FUNCTION_BLOCK Example29_recoveryaccident	//any number of flyways and xbots (real physical, with at least 1 xbot having suffered a tracking error) - GetAllAccidentXbots, RecoverAccidentXbot
VAR_INPUT
	Execute : BOOL;
END_VAR
VAR_OUTPUT
	Done : BOOL;
END_VAR
VAR_IN_OUT
	PM_Controller : PMControllerType;	// the planar motor controller to use
END_VAR
VAR
	PMC_ReadNumAccidentXbots1 : PMC_ReadNumAccidentXbots;
	PMC_GetAllAccidentXbots1 : PMC_GetAllAccidentXbots;
	PMC_RecoverAccidentXbot1 : PMC_RecoverAccidentXbot;
	xbot_index : INT := 0;
	recovering_xbots : BOOL := FALSE;
	num_accident : USINT;
END_VAR

//any number of flyways and xbots (real physical, with at least 1 xbot having suffered a tracking error) - GetAllAccidentXbots, RecoverAccidentXbot

//reset index
IF(Execute = FALSE)THEN
	xbot_index := 0;
	recovering_xbots := 0;
	Done := 0;
END_IF;

//wait until a xbot has suffered a tracking error
PMC_ReadNumAccidentXbots1(Enable := Execute,nXbots => num_accident,PM_Controller := PM_Controller);
IF(num_accident > 0)THEN
	recovering_xbots := TRUE;
END_IF;

//get IDs of all xbots that have suffered tracking errors
PMC_GetAllAccidentXbots1(Execute := recovering_xbots,PM_Controller := PM_Controller);

//recover one of the accident xbots
PMC_RecoverAccidentXbot1(Execute := PMC_GetAllAccidentXbots1.Done,XbotID := PMC_GetAllAccidentXbots1.XbotIDs[xbot_index],RecoveryMode := 0,ShortAxis := 0,PM_Controller := PM_Controller);

//reset recover_accident function block and increment the index if it is done and not all accident xbots have been recovered 
IF(PMC_RecoverAccidentXbot1.Done)THEN
	IF(xbot_index + 1 < PMC_GetAllAccidentXbots1.nXbots)THEN
		xbot_index := xbot_index + 1;
		PMC_RecoverAccidentXbot1(Execute := FALSE,XbotID := PMC_GetAllAccidentXbots1.XbotIDs[xbot_index],RecoveryMode := 0,ShortAxis := 0,PM_Controller := PM_Controller);
	ELSE
		Done := TRUE;
	END_IF;
END_IF;

END_FUNCTION_BLOCK
